(* Logix 5000 AddOnInstructionDefinition export ACS_ENABLE_DRIVE; software revision 20.01 *)

ADD_ON_INSTRUCTION ACS_ENABLE_DRIVE   (* revision 2.0, vendor Tolomatic, Inc *)
// Enable ACS Drive
VAR_IN_OUT
   DriveCMD : SINT; {required}   // ToloOutput Reference
END_VAR

ROUTINE Logic   (* ladder *)
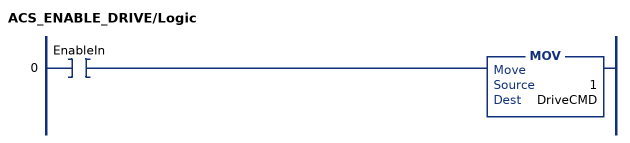
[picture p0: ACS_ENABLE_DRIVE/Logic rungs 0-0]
   0: XIC(EnableIn)MOV(1,DriveCMD);
END_ROUTINE
END_ADD_ON_INSTRUCTION
